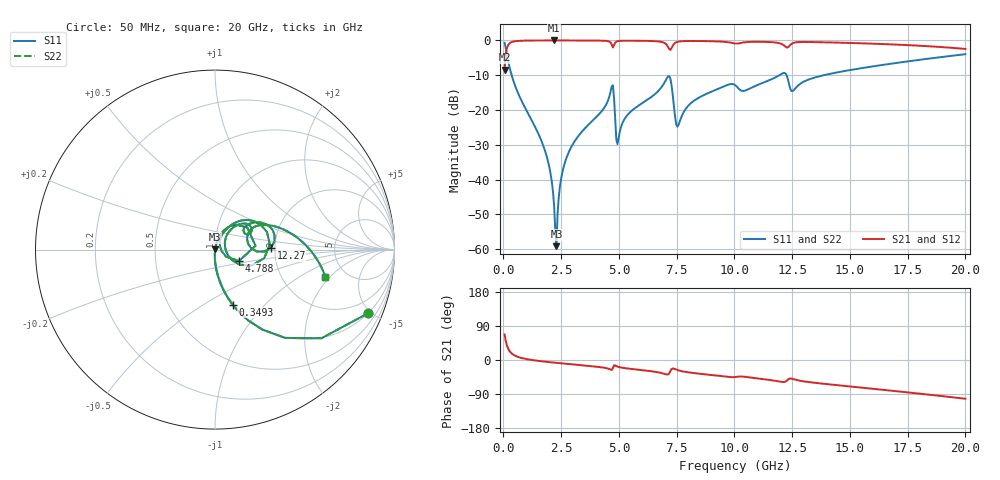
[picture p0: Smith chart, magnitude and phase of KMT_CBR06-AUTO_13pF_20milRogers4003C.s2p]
! Data measured by Modelithics Inc. support@modelithics.com 813-866-6335
! KEMET CBR06-AUTO 13pF, Pad Width= 0.851mm, Pad Length= 0.64mm, Pad Gap= 0.62mm, 20mil Rogers 4003C substrate Data, January 2022
# hz S ma R 50
! 2 Port Network Data from SP1.SP block
! freq  magS11  angS11  magS21  angS21  magS12  angS12  magS22  angS22
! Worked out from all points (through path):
!   401 points, 50 MHz to 20 GHz, reference 50 ohm
!   highest |S21| = -0.01 dB at 2.195 GHz (marker M1); lowest = -8.4 dB at 50 MHz (marker M2)
!   group delay of S21, straight-line fit = 14.8 ps
!   lowest |S11| = -59.1 dB at 2.294 GHz (marker M3), VSWR 1.00, Z = 50.1 + j0.0681 ohm
!   |S11| at or under -10 dB: 356 MHz to 11.94 GHz (11.59 GHz wide, 188 % of centre); 12.26 GHz to 13.86 GHz (1.603 GHz wide, 12.3 % of centre)
!   |S22| runs from -59.1 to -0.7 dB; largest |S21 - S12| = 0
!   S11 on the Smith chart (normalised r, x): 50 MHz: 0.99, -4.82; 349.2 MHz: 0.99, -0.68; 4.788 GHz: 1.30, -0.17; 12.27 GHz: 1.90, +0.04; 20 GHz: 3.50, -1.78
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5e7  0.9246 -22.5  0.3807 67.4  0.3807 67.4  0.9246 -22.5
3.4925e8  0.3218 -72.3  0.9464 17.6  0.9464 17.6  0.3218 -72.3
1.795625e9  0.02622 -92.9  0.9989 -4.4  0.9989 -4.4  0.02622 -92.9
2.045e9  0.01192 -92.5  0.9991 -6.0  0.9991 -6.0  0.01192 -92.5
2.194625e9  0.004201 -86.5  0.9992 -6.9  0.9992 -6.9  0.004201 -86.5
2.294375e9  0.001109 37.8  0.9991 -7.5  0.9991 -7.5  0.001109 37.8
2.6435e9  0.01687 77.5  0.9989 -9.6  0.9989 -9.6  0.01687 77.5
3.391625e9  0.04874 74.8  0.9976 -13.9  0.9976 -13.9  0.04874 74.8
4.6385e9  0.1837 49.0  0.9345 -25.3  0.9345 -25.3  0.1837 49.0
4.788125e9  0.1486 -25.0  0.8536 -14.0  0.8536 -14.0  0.1486 -25.0
4.987625e9  0.04012 48.0  0.983 -18.4  0.983 -18.4  0.04012 48.0
5.386625e9  0.08641 64.6  0.9917 -22.5  0.9917 -22.5  0.08641 64.6
6.73325e9  0.1924 52.4  0.9655 -32.9  0.9655 -32.9  0.1924 52.4
7.182125e9  0.3069 5.5  0.7456 -34.7  0.7456 -34.7  0.3069 5.5
7.581125e9  0.0613 26.5  0.9624 -27.4  0.9624 -27.4  0.0613 26.5
8.279375e9  0.1382 51.8  0.9817 -34.7  0.9817 -34.7  0.1382 51.8
1.0025e10  0.2291 26.9  0.9043 -44.9  0.9043 -44.9  0.2291 26.9
1.226938e10  0.3115 1.9  0.7925 -54.4  0.7925 -54.4  0.3115 1.9
1.251875e10  0.1872 16.6  0.9104 -50.0  0.9104 -50.0  0.1872 16.6
1.336662e10  0.2857 28.6  0.9476 -59.4  0.9476 -59.4  0.2857 28.6
1.670825e10  0.4597 8.7  0.8799 -80.4  0.8799 -80.4  0.4597 8.7
2e10  0.6341 -13.9  0.7551 -102.3  0.7551 -102.3  0.6341 -13.9
